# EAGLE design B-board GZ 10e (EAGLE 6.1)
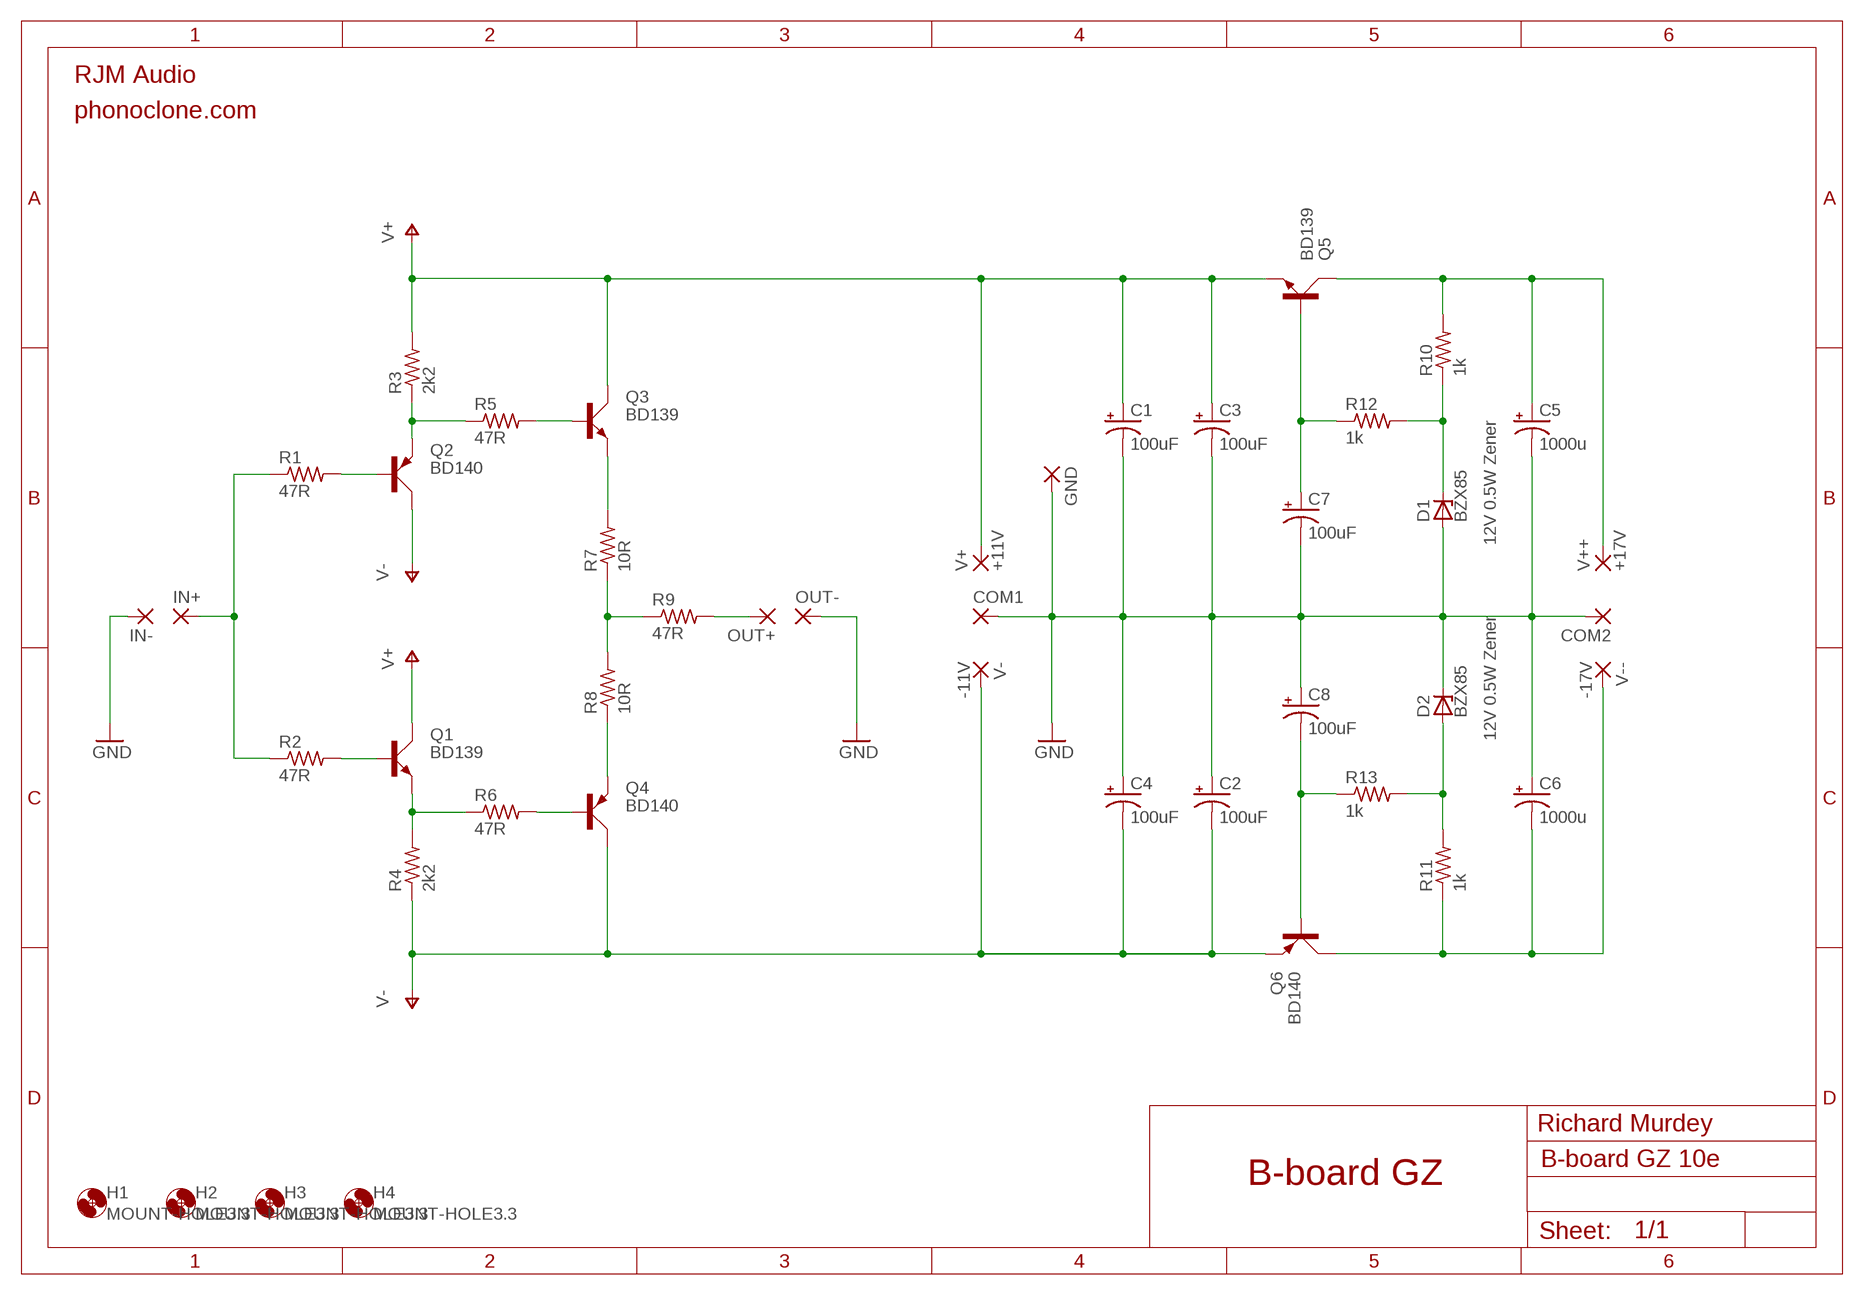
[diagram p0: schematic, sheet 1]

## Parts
C1  100uF  CPOL-USE2.5-6  [E2,5-6]
C2  100uF  CPOL-USE2.5-6  [E2,5-6]
C3  100uF  CPOL-USE2.5-6  [E2,5-6]
C4  100uF  CPOL-USE2.5-6  [E2,5-6]
C5  1000u  CPOL-USE5-10.5  [E5-10,5]
C6  1000u  CPOL-USE5-10.5  [E5-10,5]
C7  100uF  CPOL-USE2.5-6  [E2,5-6]
C8  100uF  CPOL-USE2.5-6  [E2,5-6]
COM1  2,54/1,0  [2,54/1,0]
COM2  2,54/1,0  [2,54/1,0]
D1  BZX85  [DO41Z10]
D2  BZX85  [DO41Z10]
GND  2,54/1,0  [2,54/1,0]
H1  MOUNT-HOLE3.3  [3,3]
H2  MOUNT-HOLE3.3  [3,3]
H3  MOUNT-HOLE3.3  [3,3]
H4  MOUNT-HOLE3.3  [3,3]
IN+  2,54/1,0  [2,54/1,0]
IN-  2,54/1,0  [2,54/1,0]
OUT+  2,54/1,0  [2,54/1,0]
OUT-  2,54/1,0  [2,54/1,0]
Q1  BD139  [TO126AV]
Q2  BD140  [TO126AV]
Q3  BD139  [TO126AV]
Q4  BD140  [TO126AV]
Q5  BD139  [TO126AV]
Q6  BD140  [TO126AV]
R1  47R  R-US_0309/12  [0309/12]
R2  47R  R-US_0309/12  [0309/12]
R3  2k2  R-US_0411/15  [0411/15]
R4  2k2  R-US_0411/15  [0411/15]
R5  47R  R-US_0309/12  [0309/12]
R6  47R  R-US_0309/12  [0309/12]
R7  10R  R-US_0309/12  [0309/12]
R8  10R  R-US_0309/12  [0309/12]
R9  47R  R-US_0309/12  [0309/12]
R10  1k  R-US_0309/12  [0309/12]
R11  1k  R-US_0309/12  [0309/12]
R12  1k  R-US_0309/12  [0309/12]
R13  1k  R-US_0309/12  [0309/12]
V+  +11V  2,54/1,0  [2,54/1,0]
V++  +17V  2,54/1,0  [2,54/1,0]
V-  -11V  2,54/1,0  [2,54/1,0]
V--  -17V  2,54/1,0  [2,54/1,0]

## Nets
GND: C1.- C2.+ C3.- C4.+ C5.- C6.+ C7.- C8.+ COM1.1(P) COM2.1(P) D1.A D2.C GND.1(P) IN-.1(P) OUT-.1(P)
INPUT: IN+.1(P) R1.1 R2.1
N$1: Q2.B R1.2
N$2: Q1.B R2.2
N$4: Q2.E R3.1 R5.1
N$8: Q1.E R4.2 R6.1
N$10: Q4.B R6.2
N$11: Q3.B R5.2
N$12: C8.- Q6.B R13.1
N$13: Q4.E R8.1
N$14: R7.1 R8.2 R9.1
N$15: Q3.E R7.2
N$17: C7.+ Q5.B R12.1
N$19: D2.A R11.2 R13.2
N$20: D1.C R10.1 R12.2
OUTPUT: OUT+.1(P) R9.2
V+: C1.+ C3.+ Q1.C Q3.C Q5.E R3.2 V+.1(P)
V++: C5.+ Q5.C R10.2 V++.1(P)
V-: C2.- C4.- Q2.C Q4.C Q6.E R4.1 V-.1(P)
V--: C6.- Q6.C R11.1 V--.1(P)

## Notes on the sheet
- RJM Audio
- phonoclone.com
- 12V 0.5W Zener
- 12V 0.5W Zener
- Richard Murdey
- B-board GZ

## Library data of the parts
C1-C8 = resistor:CPOL-US: POLARIZED CAPACITOR, American symbol
COM1 COM2 GND IN+ IN- OUT+ OUT- V+ V++ V- V-- = wirepad:2,54/1,0: THROUGH-HOLE PAD
D1 D2 = diode:BZX85: Z DIODE
H1-H4 = holes:MOUNT-HOLE: MOUNTING HOLE with drill center marker
Q1 Q3 Q5 = transistor-power:BD139: NPN TRANSISTOR
Q2 Q4 Q6 = transistor-power:BD140: PNP TRANSISTOR
R1-R13 = resistor:R-US_: RESISTOR, American symbol

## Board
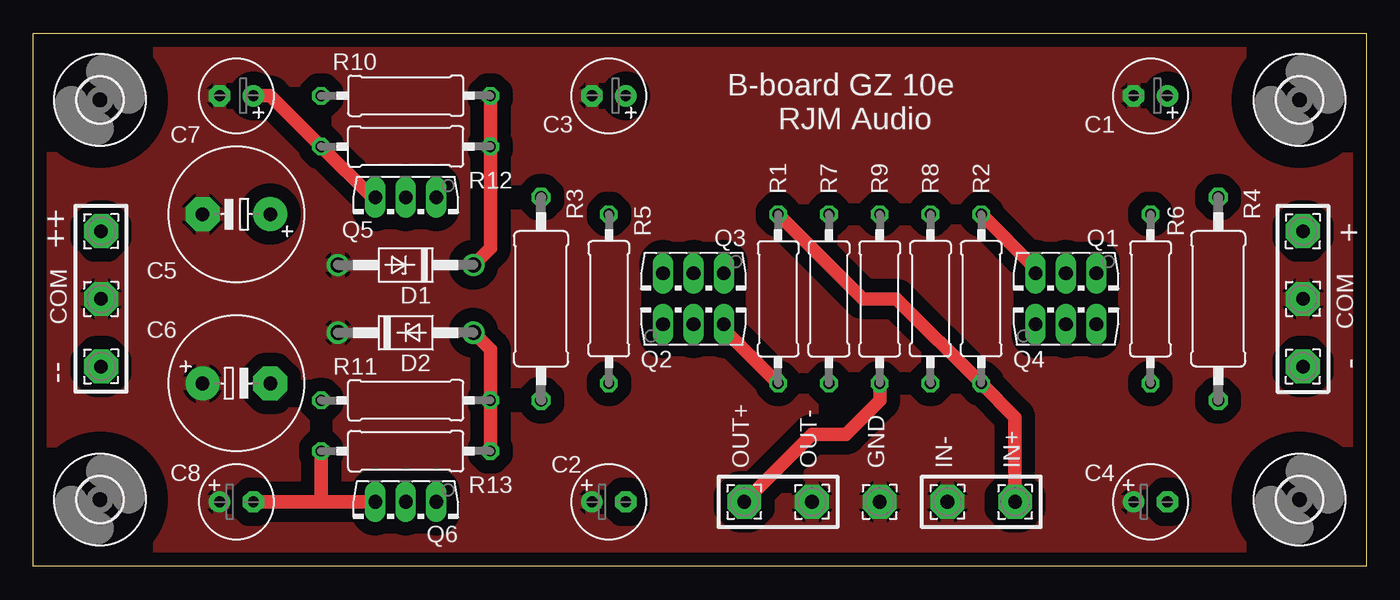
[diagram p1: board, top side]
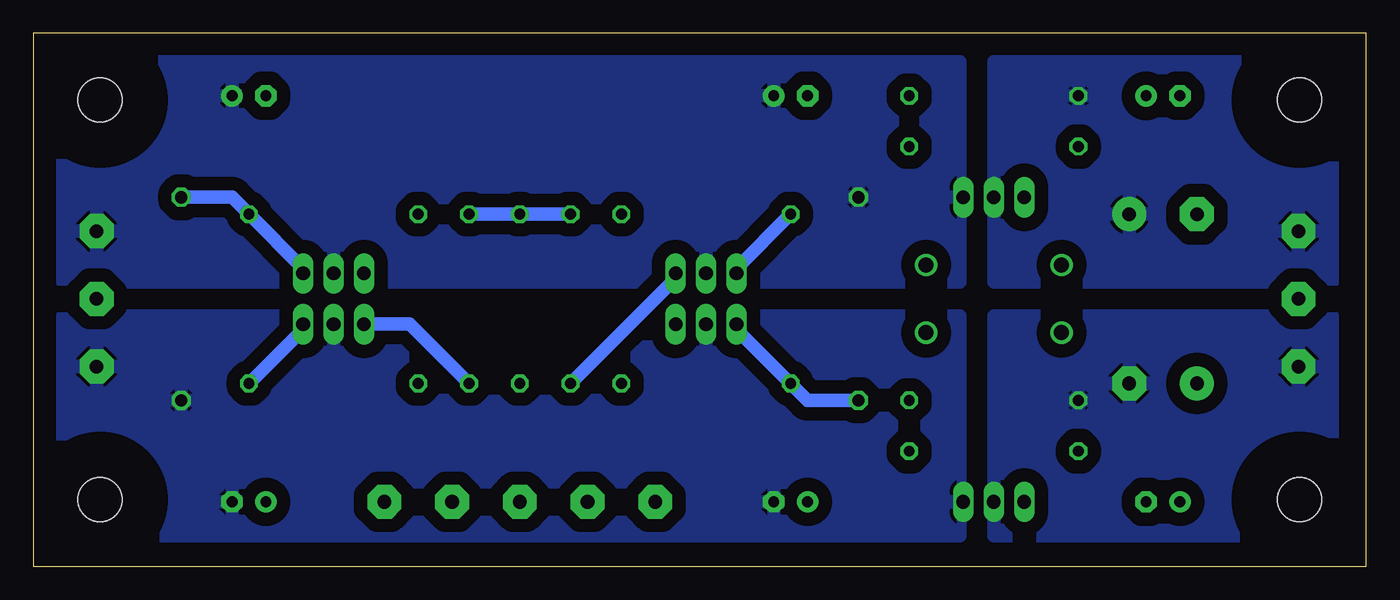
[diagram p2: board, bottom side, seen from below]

Size 100 x 40 mm. Coordinates in mm from the lower left corner, seen from the top.
Outline: 0,0 0,40 100,40 100,0 0,0
Copper layers (1*16): Top 0.035mm / dielectric 1.5mm / Bottom 0.035mm
Design rules: minimum track width 10mil, minimum drill 24mil, track to track 8mil, track to pad 8mil, pad to pad 8mil, via to via 8mil, smd to smd 8mil, copper to edge 40mil, drill to drill 8mil, minimum pad ring 10mil, minimum via ring 8mil, stop-mask expansion 4mil, vias tented up to drill 0mil, thermal gap 10mil

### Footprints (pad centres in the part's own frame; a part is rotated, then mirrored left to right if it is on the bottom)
E2,5-6 = drill 0.813 pad 1.6: + -1.27,0 | drill 0.813 pad 1.6 octagon: - 1.27,0
E5-10,5 = drill 1.016 pad 2.54: + -2.54,0 | drill 1.016 pad 2.54 octagon: - 2.54,0
2,54/1,0 = drill 1.016 pad 2.54 octagon: 1 0,0
DO41Z10 = drill 1.118: A 5.08,0; C -5.08,0
3,3 = hole 3.3: 0,0
TO126AV = drill 1.016 long: B 2.286,-1.27; C 0,-1.27; E -2.286,-1.27
0309/12 = drill 0.813 octagon: 1 -6.35,0; 2 6.35,0
0411/15 = drill 0.914 octagon: 1 -7.62,0; 2 7.62,0

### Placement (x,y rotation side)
C1  83.82,35.31 180 top
C2  43.18,4.83 0 top
C3  43.18,35.31 180 top
C4  83.82,4.83 0 top
C5  15.24,26.42 180 top
C6  15.24,13.72 0 top
C7  15.24,35.31 180 top
C8  15.24,4.83 0 top
COM1  5.08,20.07 0 top
COM2  95.25,20.07 270 top
D1  27.94,22.61 180 top
D2  27.94,17.53 0 top
GND  63.5,4.83 0 top
H1  5,5 0 top
H2  5,35 0 top
H3  95,35 0 top
H4  95,5 0 top
IN+  73.66,4.83 270 top
IN-  68.58,4.83 270 top
OUT+  53.34,4.83 270 top
OUT-  58.42,4.83 270 top
Q1  77.47,20.7 180 top
Q2  49.53,19.43 0 top
Q3  49.53,20.7 180 top
Q4  77.47,19.43 0 top
Q5  27.94,26.42 180 top
Q6  27.94,3.56 180 top
R1  55.88,20.07 270 top
R2  71.12,20.07 90 top
R3  38.1,20.07 90 top
R4  88.9,20.07 90 top
R5  43.18,20.07 90 top
R6  83.82,20.07 270 top
R7  59.69,20.07 270 top
R8  67.31,20.07 90 top
R9  63.5,20.07 270 top
R10  27.94,35.31 180 top
R11  27.94,12.45 0 top
R12  27.94,31.5 0 top
R13  27.94,8.64 0 top
V+  95.25,25.15 0 top
V++  5.08,25.15 270 top
V-  95.25,14.99 0 top
V--  5.08,14.99 270 top

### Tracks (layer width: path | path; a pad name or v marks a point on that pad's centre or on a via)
GND
  pour Top (isolate 1.016): 1.27,39.12 99.06,39.12 99.06,1.02 1.27,1.02
INPUT
  Top 1.016: R1.1 62.23,20.07 64.77,20.07 R2.1 73.66,11.18 IN+.1
N$1
  Top 1.016: R1.2 51.82,17.78 Q2.B
N$2
  Top 1.016: R2.2 75.18,22.36 Q1.B
N$4
  Bottom 1.016: R3.1 41.91,12.45 R5.1 47.24,17.78 Q2.E
N$8
  Bottom 1.016: R4.2 85.09,27.69 R6.1 79.76,22.36 Q1.E
N$10
  Bottom 1.016: R6.2 79.76,17.78 Q4.B
N$11
  Bottom 1.016: R5.2 47.24,22.36 Q3.B
N$12
  Top 1.016: C8.- 21.59,4.83 | Q6.B 21.59,4.83 | 21.59,4.83 R13.1
N$13
  Bottom 1.016: R8.1 71.75,18.16 Q4.E
N$14
  Bottom 1.016: R8.2 R9.1 R7.1
N$15
  Bottom 1.016: Q3.E 51.82,21.59 R7.2
N$17
  Top 1.016: C7.+ 17.78,35.31 R12.1 25.4,27.69 Q5.B
N$19
  Top 1.016: R13.2 R11.2 34.29,16.26 D2.A
N$20
  Top 1.016: R10.1 R12.2 34.29,23.88 D1.C
OUTPUT
  Top 1.016: R9.2 63.5,12.45 60.96,9.91 58.42,9.91 OUT+.1
V+
  pour Bottom (isolate 1.016, rank 3): 30.48,37.85 97.79,37.85 97.79,21.34 30.48,21.34
V++
  pour Bottom (isolate 1.016, rank 2): 2.54,37.85 27.94,37.85 27.94,21.34 2.54,21.34
V-
  pour Bottom (isolate 1.016, rank 3): 30.48,18.8 97.79,18.8 97.79,2.29 30.48,2.29
V--
  pour Bottom (isolate 1.016, rank 2): 27.94,18.8 2.54,18.8 2.54,2.29 27.94,2.29

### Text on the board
tPlace: + | ++ | COM | COM | - | --
tNames: B-board GZ 10e | RJM Audio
